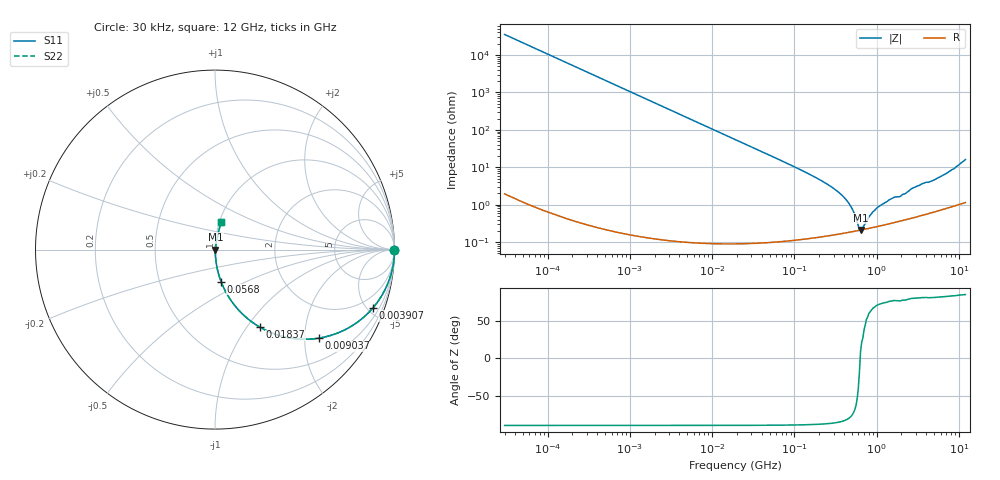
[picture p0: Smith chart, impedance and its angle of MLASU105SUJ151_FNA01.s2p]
! MLASU105SUJ151_FNA01  S-PARAMETER MODEL  ( General Type )
! Model Generated by TAIYO YUDEN Corporation (http://www.ty-top.com)
! Version 3.0
! TAIYO YUDEN Control No. 120810
! Copyright(c) 2003 TAIYO YUDEN CO.,LTD. All Rights Reserved.
! Product Description (link to TY-COMPAS)
! https://ds.yuden.co.jp/TYCOMPAS/or/detail?pn=MLASU105SUJ151JFNA01&u=M
! Products Name : Multilayer Ceramic Capacitors
! Characteristics :
!  Capacitance : 150 pF , Rated Voltage : 50V , TCC : UJ / U2J
!  Case Size : 1.0 x 0.5 / 0.039 x 0.02 [mm/inch] , Thickness : 0.5 / 0.02 [mm/inch]
!  (Conditions: Temperature = 25 degC , DC Bias Current/Voltage = 0A / 0V)
! External Node Assignments :
!  1  o---| |---o  2
! GND o---------o GND
! Frequency Range : 0.03MHz  -  12000MHz  [ 401 STEP ]
# MHz S RI R 50
! Freq[MHz].  S11 Real  S11 Imag  S21 Real  S21 Imag  S12 Real  S12 Imag  S22 Real  S22 Imag
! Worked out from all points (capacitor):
!   401 points, 30 kHz to 12 GHz, reference 50 ohm
!   read as one part in series: C = 150 pF near 32 kHz
!   lowest |Z| = 214 mohm at 637.8 MHz (marker M1)
!   series resonance near 631.1 MHz, so ESL is about 420 pH
!   S11 on the Smith chart (normalised r, x): 30 kHz: open; 3.907 MHz: 1.00, -5.41; 9.037 MHz: 1.00, -2.34; 18.37 MHz: 1.00, -1.15; 56.8 MHz: 1.00, -0.37; 12 GHz: 1.02, +0.32
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0.03  1 -0.00284  8.2e-06 0.00284  8.2e-06 0.00284  1 -0.00284
0.260295  0.9994 -0.0246  0.000607 0.0246  0.000607 0.0246  0.9994 -0.0246
0.886466  0.993 -0.0832  0.00699 0.0832  0.00699 0.0832  0.993 -0.0832
2.258455  0.9564 -0.2042  0.0436 0.2042  0.0436 0.2042  0.9564 -0.2042
3.907499  0.8798 -0.325  0.1202 0.325  0.1202 0.325  0.8798 -0.325
9.037177  0.5779 -0.4935  0.4221 0.4935  0.4221 0.4935  0.5779 -0.4935
18.37156  0.249 -0.4316  0.751 0.4316  0.751 0.4316  0.249 -0.4316
18.97367  0.2371 -0.4245  0.7629 0.4245  0.7629 0.4245  0.2371 -0.4245
30.77716  0.1058 -0.3063  0.8942 0.3063  0.8942 0.3063  0.1058 -0.3063
56.79713  0.0339 -0.1783  0.9661 0.1783  0.9661 0.1783  0.0339 -0.1783
164.6252  0.00484 -0.0595  0.9952 0.0595  0.9952 0.0595  0.00484 -0.0595
284.8288  0.00239 -0.0294  0.9976 0.0294  0.9976 0.0294  0.00239 -0.0294
406.107  0.00197 -0.0152  0.998 0.0152  0.998 0.0152  0.00197 -0.0152
492.8008  0.00195 -0.00832  0.998 0.00832  0.998 0.00832  0.00195 -0.00832
598.0015  0.00205 -0.00177  0.998 0.00177  0.998 0.00177  0.00205 -0.00177
637.8412  0.0021 0.000351  0.9979 -0.000351  0.9979 -0.000351  0.0021 0.000351
680.3351  0.00216 0.00113  0.9978 -0.00113  0.9978 -0.00113  0.00216 0.00113
939.2353  0.00255 0.00647  0.9974 -0.00647  0.9974 -0.00647  0.00255 0.00647
1428.372  0.00327 0.0131  0.9967 -0.0131  0.9967 -0.0131  0.00327 0.0131
2903.719  0.00539 0.0286  0.9946 -0.0286  0.9946 -0.0286  0.00539 0.0286
5358.614  0.00903 0.0488  0.991 -0.0488  0.991 -0.0488  0.00903 0.0488
12000  0.0356 0.153  0.9644 -0.153  0.9644 -0.153  0.0356 0.153
